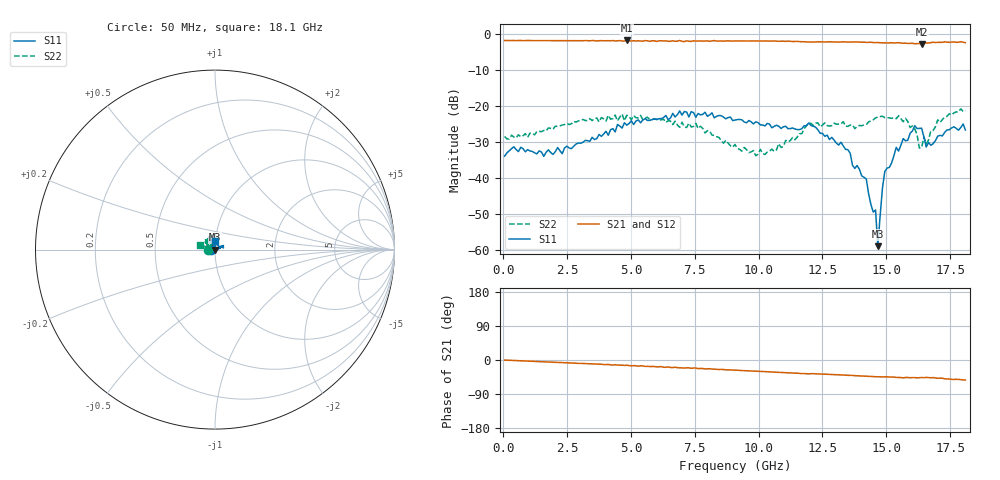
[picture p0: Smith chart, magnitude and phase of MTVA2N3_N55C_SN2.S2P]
! Network Analyzer HP8720D.06.14 Serial No. US36140669
! 11 May 2005  12:41:39
! Frequency  S11  S21  S12  S22
# HZ  S  DB R 50
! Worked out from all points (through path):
!   201 points, 50 MHz to 18.1 GHz, reference 50 ohm
!   highest |S21| = -1.92 dB at 4.833 GHz (marker M1); lowest = -2.9 dB at 16.39 GHz (marker M2)
!   group delay of S21, straight-line fit = 8.09 ps
!   lowest |S11| = -59.0 dB at 14.67 GHz (marker M3), VSWR 1.00, Z = 50.1 + j0.0309 ohm
!   |S11| at or under -10 dB: start of sweep to end of sweep
!   |S22| runs from -33.9 to -20.9 dB; largest |S21 - S12| = 0.024
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5e7  -34.05 -175.4  -1.94 -0.3  -1.97 -0.7  -28.60 -175.9
3.1185e9  -30.20 104.8  -1.99 -9.2  -1.99 -9.9  -23.87 143.2
4.83325e9  -25.45 94.8  -1.92 -13.9  -1.94 -15.2  -22.71 123.2
6.09675e9  -23.65 96.4  -2.03 -17.9  -1.97 -18.2  -24.10 121.4
7.54075e9  -23.23 97.6  -2.10 -21.2  -1.94 -22.6  -24.94 123.7
9.075e9  -24.01 130.8  -2.05 -26.8  -2.04 -27.3  -30.80 146.9
1.024825e10  -25.66 139.1  -2.05 -30.7  -2.05 -31.2  -33.58 157.9
1.21435e10  -25.74 131.8  -2.35 -35.9  -2.32 -36.5  -25.56 135.1
1.32265e10  -30.18 109.8  -2.34 -39.4  -2.34 -39.9  -25.07 123.4
1.421925e10  -40.44 54.5  -2.47 -42.6  -2.45 -43.2  -25.28 146.0
1.439975e10  -47.48 14.6  -2.42 -43.4  -2.40 -43.7  -24.24 141.9
1.458025e10  -48.98 -29.2  -2.52 -44.2  -2.42 -44.8  -23.42 143.2
1.46705e10  -59.04 16.0  -2.49 -44.1  -2.48 -44.5  -23.19 139.8
1.494125e10  -38.33 37.6  -2.57 -44.4  -2.61 -44.5  -23.36 134.4
1.512175e10  -37.15 25.7  -2.59 -45.0  -2.50 -45.1  -23.40 129.0
1.53925e10  -31.60 23.8  -2.59 -46.0  -2.51 -45.8  -23.64 124.1
1.57535e10  -29.78 28.6  -2.67 -46.2  -2.79 -47.6  -23.54 108.4
1.638525e10  -26.29 12.4  -2.88 -46.3  -2.73 -46.6  -31.69 117.3
1.64755e10  -28.75 23.5  -2.75 -46.6  -2.86 -46.3  -28.76 128.8
1.656575e10  -31.50 19.3  -2.61 -45.9  -2.60 -46.6  -30.62 152.7
1.7017e10  -28.50 71.9  -2.45 -48.3  -2.48 -49.3  -23.96 164.4
1.81e10  -26.77 86.9  -2.54 -52.9  -2.49 -54.6  -21.34 162.8
